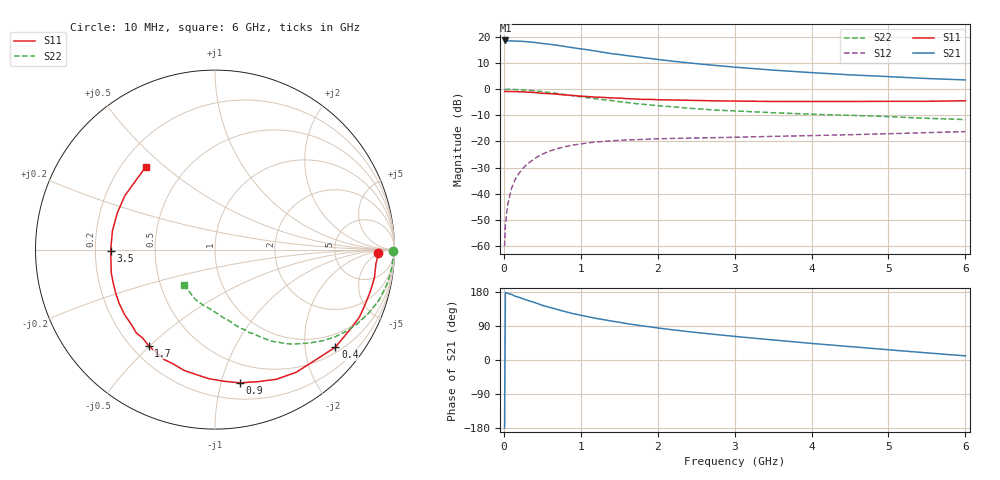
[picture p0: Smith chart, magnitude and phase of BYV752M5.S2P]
! SIEMENS Small Signal Semiconductors
! BFY420
! Si NPN RF SIEGET Grounded Emitter Transistor in MICRO-X
! VCE = 0.75 V  IC = 2.5 mA
! Common Emitter S-Parameters:  October  1996
# GHz  S  MA  R  50
!  f  S11  S21  S12  S22
! GHz  MAG  ANG  MAG  ANG  MAG  ANG  MAG  ANG
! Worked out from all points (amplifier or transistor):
!   36 points, 10 MHz to 6 GHz, reference 50 ohm
!   highest |S21| = 18.6 dB at 20 MHz (marker M1)
!   |S21| within 3 dB of that: start of sweep to 950 MHz
!   unconditionally stable (mu >= 1): 3.723 GHz to end of sweep
!   at 250 MHz: K = 0.06, MSG = 24.2 dB, |S12| = -30.2 dB
!   at 1.4 GHz: K = 0.37, MSG = 16.7 dB, |S12| = -19.8 dB
!   at 6 GHz: K = 1.25, MAG = 6.9 dB, |S12| = -16.2 dB
!   S11 on the Smith chart (normalised r, x): 10 MHz: 19, -4; 400 MHz: 0.63, -2.69; 900 MHz: 0.33, -1.15; 1.7 GHz: 0.27, -0.49; 3.5 GHz: 0.26, -0.00; 6 GHz: 0.30, +0.43
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0.01  0.9063 -1.2  8.512 -179.6  0.001 95.6  0.9929 -0.5
0.02  0.9068 -2.5  8.515 178.2  0.0026 93.4  0.9856 -1.1
0.05  0.9001 -5.0  8.35 175.8  0.0062 88.4  0.9924 -3.0
0.1  0.902 -10.0  8.367 173.0  0.0128 84.3  0.9895 -5.9
0.15  0.8962 -15.0  8.265 168.2  0.0192 80.4  0.9832 -8.8
0.25  0.8884 -24.9  8.173 161.4  0.031 75.4  0.9657 -14.4
0.4  0.8633 -39.0  7.804 151.7  0.0473 67.7  0.9259 -22.5
0.5  0.8315 -47.8  7.459 144.3  0.0572 62.3  0.8941 -27.6
0.6  0.8194 -56.5  7.175 138.7  0.066 58.3  0.8599 -32.1
0.7  0.7993 -64.7  6.86 133.0  0.0732 53.7  0.8237 -36.4
0.9  0.7552 -79.4  6.178 122.4  0.0857 45.8  0.7495 -43.7
1.1  0.72 -92.8  5.621 113.9  0.0944 40.1  0.6847 -50.2
1.2  0.7034 -98.9  5.317 109.8  0.0979 37.4  0.6557 -53.1
1.4  0.6787 -109.8  4.765 102.7  0.1029 32.9  0.6047 -57.8
1.7  0.6508 -124.7  4.199 93.1  0.108 27.7  0.532 -63.9
2  0.6275 -137.2  3.695 84.6  0.1126 23.6  0.4826 -68.9
2.2  0.6203 -144.4  3.41 79.6  0.1145 21.4  0.4596 -72.1
2.8  0.5967 -162.1  2.796 66.4  0.1188 17.1  0.3941 -80.3
3.5  0.5814 -179.5  2.309 52.9  0.1253 13.9  0.3542 -88.5
4.5  0.5813 159.3  1.876 35.4  0.1347 10.1  0.3165 -102.0
5.5  0.5855 139.1  1.596 18.8  0.1477 6.5  0.2772 -120.3
6  0.6006 129.9  1.501 10.9  0.1544 4.8  0.2625 -131.2
